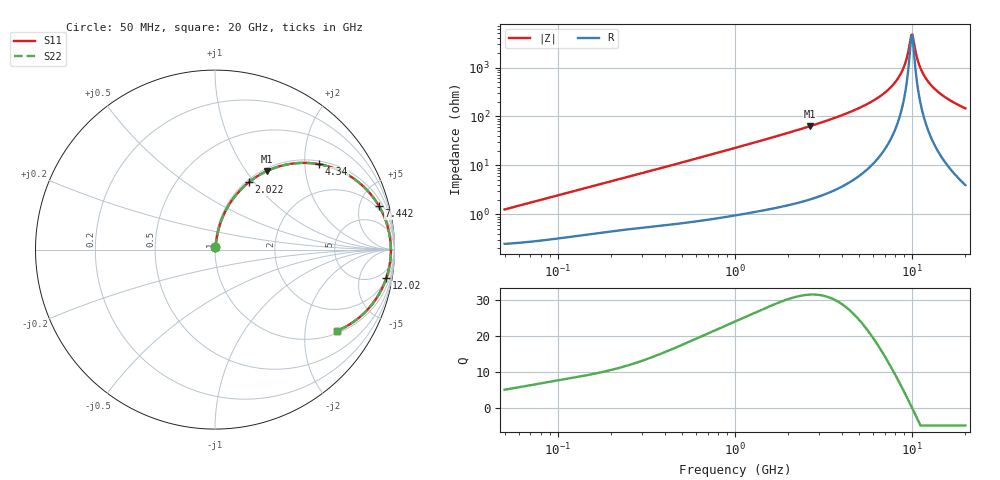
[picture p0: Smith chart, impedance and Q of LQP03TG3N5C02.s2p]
!Murata Part Number: LQP03TG3N5C02
!These Parameters are Measured in Series Mode Connection
!  o--[Z]--o
!Port1  Port2
!  o-------o
!Freq. Start=50[MHz] Stop=20[GHz], 401[Steps]
# Hz S RI R 50
!Freq.(Hz) S11(Real) S11(Imag) S21(Real) S21(Imag) S12(Real) S12(Imag) S22(Real) S22(Imag)
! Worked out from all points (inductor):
!   401 points, 50 MHz to 20 GHz, reference 50 ohm
!   read as one part in series: L = 3.9 nH near 51.52 MHz
!   highest Q = 31.5 at 2.647 GHz (marker M1), where L = 3.79 nH
!   self-resonance near 9.892 GHz
!   S11 on the Smith chart (normalised r, x): 50 MHz: 1.00, +0.02; 2.022 GHz: 1.03, +0.94; 4.34 GHz: 1.09, +2.36; 7.442 GHz: 1.61, +7.36; 12.02 GHz: 2, -12; 20 GHz: 1.08, -2.93
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5e7  0.00262 0.0123  0.9974 -0.0123  0.9974 -0.0123  0.00262 0.0123
1.364002e8  0.00476 0.0323  0.9952 -0.0323  0.9952 -0.0323  0.00476 0.0323
3.721004e8  0.0129 0.0838  0.9871 -0.0838  0.9871 -0.0838  0.0129 0.0838
1e9  0.057 0.2119  0.943 -0.2119  0.943 -0.2119  0.057 0.2119
2.021818e9  0.188 0.3746  0.812 -0.3746  0.812 -0.3746  0.188 0.3746
2.647493e9  0.291 0.4386  0.709 -0.4386  0.709 -0.4386  0.291 0.4386
2.728004e9  0.3049 0.4448  0.6951 -0.4448  0.6951 -0.4448  0.3049 0.4448
4.34015e9  0.5805 0.4757  0.4195 -0.4757  0.4195 -0.4757  0.5805 0.4757
5.944466e9  0.7936 0.3803  0.2064 -0.3803  0.2064 -0.3803  0.7936 0.3803
7.442007e9  0.9144 0.2414  0.0856 -0.2414  0.0856 -0.2414  0.9144 0.2414
8.141811e9  0.9475 0.1724  0.0525 -0.1724  0.0525 -0.1724  0.9475 0.1724
8.774992e9  0.9667 0.1107  0.0333 -0.1107  0.0333 -0.1107  0.9667 0.1107
9.178299e9  0.9742 0.0725  0.0258 -0.0725  0.0258 -0.0725  0.9742 0.0725
9.745021e9  0.9795 0.0206  0.0205 -0.0206  0.0205 -0.0206  0.9795 0.0206
9.892087e9  0.98 0.00759  0.02 -0.00759  0.02 -0.00759  0.98 0.00759
1.019291e10  0.9798 -0.0185  0.0202 0.0185  0.0202 0.0185  0.9798 -0.0185
1.066139e10  0.977 -0.0576  0.023 0.0576  0.023 0.0576  0.977 -0.0576
1.115139e10  0.971 -0.0962  0.029 0.0962  0.029 0.0962  0.971 -0.0962
1.201863e10  0.9543 -0.1589  0.0457 0.1589  0.0457 0.1589  0.9543 -0.1589
1.314879e10  0.9239 -0.2299  0.0761 0.2299  0.0761 0.2299  0.9239 -0.2299
1.482269e10  0.8678 -0.3139  0.1322 0.3139  0.1322 0.3139  0.8678 -0.3139
2e10  0.6771 -0.4542  0.3229 0.4542  0.3229 0.4542  0.6771 -0.4542
